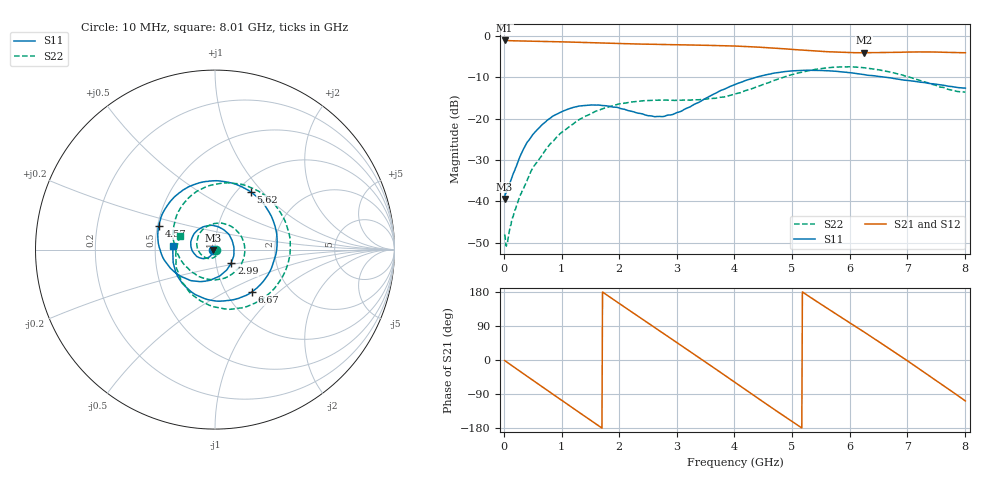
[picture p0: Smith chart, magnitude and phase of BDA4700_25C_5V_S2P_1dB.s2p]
!Agilent Technologies,E5071B,MY42404982,A.09.10
!Date: Mon Oct 20 13:26:26 2025
!Data & Calibration Information:
!Freq	S11:SOLT2(ON)	S21:SOLT2(ON)	S12:SOLT2(ON)	S22:SOLT2(ON)
# Hz S RI R 50
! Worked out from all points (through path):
!   801 points, 10 MHz to 8.01 GHz, reference 50 ohm
!   highest |S21| = -1.12 dB at 10 MHz (marker M1); lowest = -4.1 dB at 6.25 GHz (marker M2)
!   group delay of S21, straight-line fit = 286 ps
!   lowest |S11| = -39.4 dB at 10 MHz (marker M3), VSWR 1.02, Z = 49 - j0.221 ohm
!   |S11| at or under -10 dB: start of sweep to 4.38 GHz; 6.616 GHz to end of sweep
!   |S22| runs from -50.8 to -7.5 dB; largest |S21 - S12| = 0.0067
!   S11 on the Smith chart (normalised r, x): 10 MHz: 0.98, -0.00; 2.99 GHz: 1.19, -0.18; 4.57 GHz: 0.51, +0.15; 5.62 GHz: 1.15, +0.86; 6.67 GHz: 1.32, -0.69; 8.01 GHz: 0.62, +0.03
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1e7  -0.0104 -0.00225  0.8785 -0.0189  0.8788 -0.0195  0.00386 -0.000968
3.7e8  -0.0281 -0.038  0.6654 -0.5522  0.6647 -0.5526  0.0134 -0.00853
7.2e8  -0.0776 -0.0483  0.1957 -0.8312  0.196 -0.8313  -0.00228 -0.0418
1.02e9  -0.1218 -0.015  -0.2655 -0.8016  -0.2662 -0.8019  -0.0531 -0.0449
1.35e9  -0.1319 0.0541  -0.6653 -0.5008  -0.6659 -0.501  -0.0998 0.0152
1.64e9  -0.0942 0.1112  -0.816 -0.0946  -0.8162 -0.0949  -0.0816 0.0958
1.93e9  -0.0261 0.1348  -0.7426 0.3236  -0.7428 0.324  0.000711 0.1457
2.32e9  0.0644 0.0965  -0.3512 0.7146  -0.3512 0.7154  0.1293 0.0972
2.68e9  0.1051 0.0129  0.1487 0.7731  0.1487 0.7733  0.1636 -0.0339
2.99e9  0.091 -0.0738  0.5309 0.5709  0.5301 0.5707  0.1022 -0.1305
3.49e9  -0.0297 -0.1713  0.7659 -0.0641  0.766 -0.0647  -0.062 -0.1599
4.01e9  -0.2257 -0.1248  0.386 -0.6453  0.3867 -0.6449  -0.1876 -0.0624
4.57e9  -0.3137 0.1314  -0.3359 -0.6358  -0.3349 -0.6368  -0.2267 0.1439
4.97e9  -0.1877 0.3246  -0.6426 -0.2452  -0.6435 -0.2463  -0.1143 0.3153
5.35e9  0.037 0.381  -0.6289 0.1998  -0.63 0.1983  0.1132 0.3678
5.62e9  0.1989 0.3217  -0.4595 0.4494  -0.4597 0.4502  0.2813 0.2993
6.25e9  0.3391 -0.0263  0.1715 0.5987  0.1774 0.5976  0.3962 -0.1078
6.67e9  0.2065 -0.2352  0.5346 0.3318  0.5356 0.3314  0.2065 -0.3051
6.68e9  0.2018 -0.2386  0.5404 0.3224  0.5422 0.3221  0.2001 -0.3078
7.25e9  -0.0953 -0.2568  0.5643 -0.2987  0.5643 -0.2999  -0.1157 -0.2598
7.64e9  -0.2184 -0.1272  0.2268 -0.5902  0.2262 -0.5913  -0.2171 -0.0945
8.01e9  -0.2324 0.0203  -0.1939 -0.5929  -0.1933 -0.594  -0.1954 0.074
